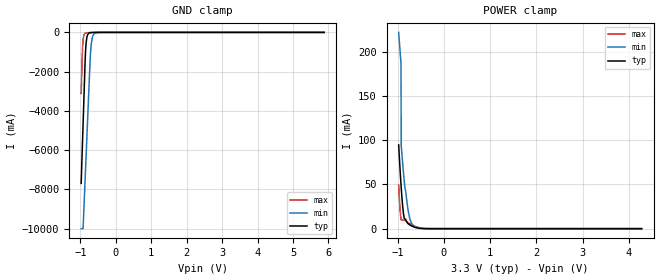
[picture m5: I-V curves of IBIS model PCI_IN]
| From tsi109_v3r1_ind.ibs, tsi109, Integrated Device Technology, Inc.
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|   MODEL PCI_IN
[Model]   PCI_IN
Model_type  Input
C_comp 4.536p 4.202p 4.874p
Polarity   Non-Inverting
Enable   Active-High
Vinl =   0.80V
Vinh =   2.00V
[Temperature Range]   27.0   125.0   -40.0
[POWER Clamp Reference]   3.30V   3.00V   3.60V
[GND Clamp Reference]   0.00V   0.00V   0.00V
[Voltage Range] 3.3 3. 3.6
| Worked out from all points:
|   GND clamp passes 1 mA (typ) near -0.58 V on its own axis
|   POWER clamp passes 1 mA (typ) near -0.59 V on its own axis
[GND Clamp]
-976.9mV  -7.694A    -10A       -3.11A
-940.4mV  -5.645A    -10A       -848.5mA
-923.3mV  -4.682A    -10A       -400.9mA
-899.6mV  -3.359A    -8.991A    -148.3mA
-863.2mV  -1.353A    -7.407A    -43.18mA
-837.4mV  -553.5mA   -6.29A     -25.04mA
-794.5mV  -126.9mA   -4.431A    -15.74mA
-727.9mV  -18.49mA   -1.562A    -9.993mA
-708.6mV  -11.57mA   -935.5mA   -8.672mA
-670mV    -5.111mA   -330.6mA   -6.269mA
-603.5mV  -1.592mA   -60.06mA   -2.971mA
5.879V    0A         0A         0A
[Power Clamp]
-976.9mV  94.83mA    222.1mA    49.21mA
-949.3mV  68.95mA    202.6mA    23.59mA
-927.1mV  50.38mA    187.5mA    11.34mA
-921.6mV  46.09mA    93.87mA    10.01mA
-888.4mV  24.44mA    72.65mA    9.649mA
-855.2mV  11.42mA    53.18mA    9.29mA
-783.3mV  6.267mA    24.59mA    7.167mA
-750.1mV  4.693mA    14.57mA    6.03mA
-705.8mV  3.303mA    6.993mA    4.715mA
-656.1mV  2.103mA    3.495mA    3.408mA
-357.3mV  8.391uA    72.94uA    14.41uA
4.277V    0A         0A         0A
